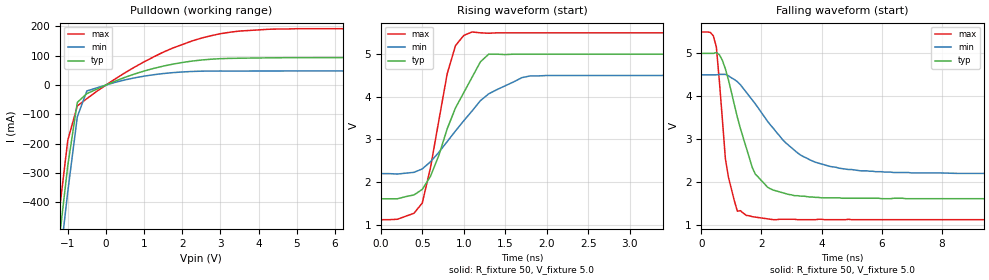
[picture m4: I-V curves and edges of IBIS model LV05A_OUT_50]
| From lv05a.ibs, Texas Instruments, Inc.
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|   Model LV05A_OUT_50
[Model]   LV05A_OUT_50
Model_type  Open_drain
Polarity   Non-Inverting
Vmeas = 2.50v
Cref = 15pf
| variable   typ   min   max
C_comp   3.34pf   2.50pf   4.18pf
[Temperature Range]   25   85   -40
[Voltage Range]   5.0   4.5   5.5
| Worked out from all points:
|   slope of the pulldown table from 0 to 0.75 V, typ, clamps not added: 19.9 ohm
|   rising waveform, R_fixture 50, V_fixture 5.0: 20-80 % time 431ps typ, 599ps min, 255ps max; typ from 1.61 V to 5 V
|   falling waveform, R_fixture 50, V_fixture 5.0: 20-80 % time 805ps typ, 1.68ns min, 378ps max; typ from 5 V to 1.61 V
[Pulldown]
|   Voltage   I(typ)   I(min)   I(max)
-5V       -5.14A     -5.22A     -5.05A
-1.5V     -853mA     -945mA     -756mA
-1.25V    -557mA     -649mA     -461mA
-1V       -274mA     -363mA     -188mA
-750mV    -58.9mA    -108mA     -71.3mA
-500mV    -29.2mA    -20mA      -46.2mA
250mV     13.9mA     9.48mA     21.5mA
1V        47.8mA     30.4mA     79.2mA
2.25V     81.6mA     46.3mA     150mA
3.25V     90.9mA     47.8mA     180mA
4.25V     92.7mA     47.9mA     190mA
10V       94.2mA     48.5mA     194mA
[Ramp]
| variable   typ   min   max
dV/dt_r   2.17E-02/1.32E-10   1.24E-02/2.60E-10   3.05E-02/1.20E-10
dV/dt_f   2.04E+00/8.07E-10   1.39E+00/1.67E-09   2.63E+00/3.15E-10
R_load = 50
[Rising Waveform]
R_fixture = 50
V_fixture = 5.0
V_fixture_min = 4.5
V_fixture_max = 5.5
|   Time   V(typ)   V(min)   V(max)
0s        1.61V      2.2V       1.12V
400ps     1.7V       2.23V      1.27V
500ps     1.83V      2.31V      1.51V
600ps     2.14V      2.48V      2.35V
800ps     3.25V      2.95V      4.54V
900ps     3.74V      3.2V       5.2V
1.1ns     4.46V      3.67V      5.52V
1.3ns     5V         4.07V      5.49V
2ns       5V         4.5V       5.5V
25ns      5V         4.5V       5.5V
[Falling Waveform]
R_fixture = 50
V_fixture = 5.0
V_fixture_min = 4.5
V_fixture_max = 5.5
|   Time   V(typ)   V(min)   V(max)
0s        5V         4.5V       5.5V
500ps     5.02V      4.5V       5.15V
800ps     4.64V      4.51V      2.55V
900ps     4.39V      4.48V      2.12V
1.2ns     3.51V      4.34V      1.32V
1.5ns     2.79V      4.09V      1.22V
2.3ns     1.84V      3.33V      1.13V
3.4ns     1.67V      2.59V      1.12V
4.9ns     1.62V      2.29V      1.13V
25ns      1.61V      2.2V       1.12V
